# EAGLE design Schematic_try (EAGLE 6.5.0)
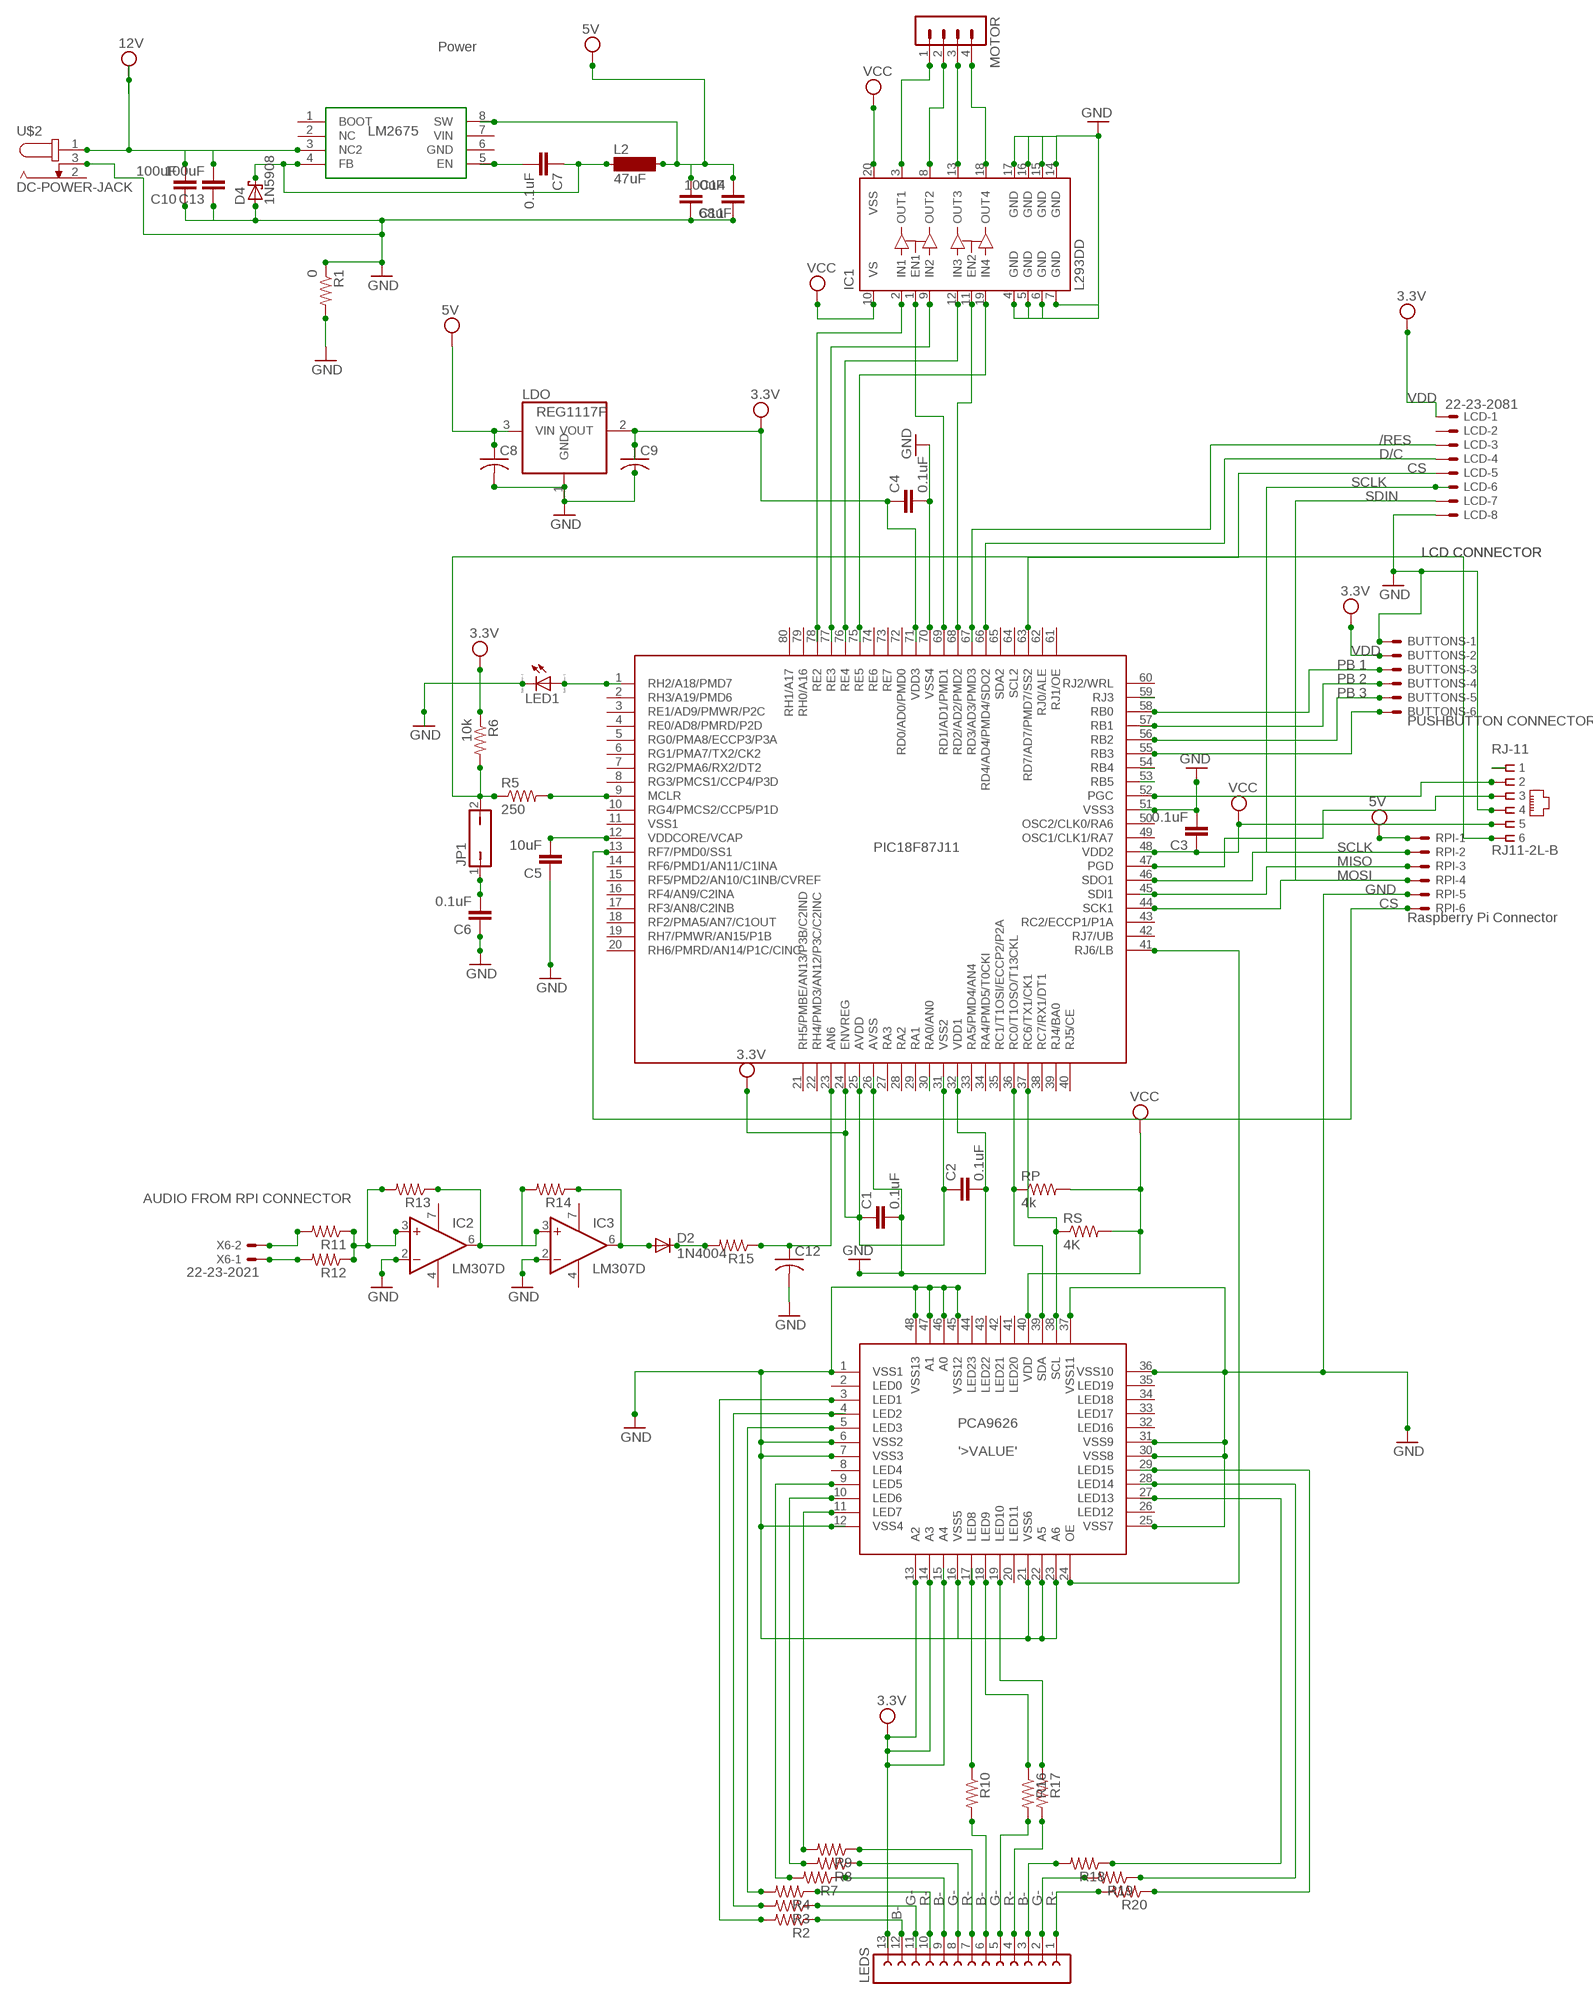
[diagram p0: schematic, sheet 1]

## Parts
BUTTONS  22-23-2061  [22-23-2061]
C1  0.1uF  C-EUC1206  [C1206]
C2  0.1uF  C-EUC1206  [C1206]
C3  0.1uF  C-EUC1206  [C1206]
C4  0.1uF  C-EUC1206  [C1206]
C5  10uF  C-EUC1206  [C1206]
C6  0.1uF  C-EUC1206  [C1206]
C7  0.1uF  C-EUC1206  [C1206]
C8  C-USC1206  [C1206]
C9  C-USC1206  [C1206]
C10  100uF  C-EUC1206  [C1206]
C11  100uF  C-EUC1206  [C1206]
C12  C-USC1206  [C1206]
C13  100uF  C-EUC1206  [C1206]
C14  68uF  C-EUC1206  [C1206]
D2  1N4004  [DO41-10]
D4  1N5908  [C4111-15]
IC1  L293DD  [SO20]
IC2  LM307D  [SO08]
IC3  LM307D  [SO08]
JP1  JP1Q  [JP1]
L2  47uF  SM-1206  [SM-1206]
LCD  22-23-2081  [22-23-2081]
LDO  REG1117F  [DD-3]
LED1  LED_E  [LED_1206]
LED_DRIVER  PCA9626  [SO-48/DIP]
LEDS  FE13-1  [FE13]
MOTOR  MA04-1  [MA04-1]
R1  0  R-US_R1206  [R1206]
R2  R-US_R1206  [R1206]
R3  R-US_R1206  [R1206]
R4  R-US_R1206  [R1206]
R5  250  R-US_R1206  [R1206]
R6  10k  R-US_R1206  [R1206]
R7  R-US_R1206  [R1206]
R8  R-US_R1206  [R1206]
R9  R-US_R1206  [R1206]
R10  R-US_R1206  [R1206]
R11  R-US_R1206  [R1206]
R12  R-US_R1206  [R1206]
R13  R-US_R1206  [R1206]
R14  R-US_R1206  [R1206]
R15  R-US_R1206  [R1206]
R16  R-US_R1206  [R1206]
R17  R-US_R1206  [R1206]
R18  R-US_R1206  [R1206]
R19  R-US_R1206  [R1206]
R20  R-US_R1206  [R1206]
RJ-11  RJ11-2L-B  [RJ11-NO_SHIELD]
RP  4k  R-US_R1206  [R1206]
RPI  22-23-2061  [22-23-2061]
RS  4K  R-US_R1206  [R1206]
U$1  PIC18F87J11  [S0-80/DIP]
U$2  DC-POWER-JACK  [PJ-036BH-SMT]
U$4  LM265  [8PIN]
X6  22-23-2021  [22-23-2021]

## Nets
+3.3: BUTTONS.2 C1.1 C2.1 C3.1 C4.1 C9.1 LCD.1 LDO.2(VOUT) LED_DRIVER.13(A2) LED_DRIVER.14(A3) LED_DRIVER.15(A4) LED_DRIVER.40(VDD) LEDS.13 R6.1 RJ-11.5 RP.2 RS.2 U$1.24(ENVREG) U$1.25(AVDD) U$1.31(VSS2) U$1.48(VDD2) U$1.71(VDD3) ; supply symbol labelled 3.3V, VCC
+5: C8.1 C11.2 C14.1 IC1.20(VSS) L2.2 LDO.3(VIN) RPI.1 U$4.8(SW) ; supply symbol labelled 5V, VCC
+12: C10.2 C13.2 IC1.10(VS) U$2.1 U$4.3(NC2) ; supply symbol labelled 12V, VCC
AGND: C12.2 IC2.2(-IN) IC3.2(-IN) R1.2 ; supply symbol labelled GND
GND: BUTTONS.1 C1.2 C2.2 C3.2 C4.2 C5.1 C6.1 C8.2 C10.1 C11.1 C13.1 C14.2 D4.A IC1.4(GND) IC1.5(GND) IC1.6(GND) IC1.7(GND) IC1.14(GND) IC1.15(GND) IC1.16(GND) IC1.17(GND) LCD.8 LDO.1(GND) LED1.C LED_DRIVER.1(VSS1) LED_DRIVER.6(VSS2) LED_DRIVER.7(VSS3) LED_DRIVER.12(VSS4) LED_DRIVER.16(VSS5) LED_DRIVER.21(VSS6) LED_DRIVER.22(A5) LED_DRIVER.23(A6) LED_DRIVER.25(VSS7) LED_DRIVER.30(VSS8) LED_DRIVER.31(VSS9) LED_DRIVER.36(VSS10) LED_DRIVER.37(VSS11) LED_DRIVER.45(VSS12) LED_DRIVER.46(A0) LED_DRIVER.47(A1) LED_DRIVER.48(VSS13) R1.1 RJ-11.4 RPI.5 U$1.26(AVSS) U$1.32(VDD1) U$1.51(VSS3) U$1.70(VSS4) U$2.3
N$1: LCD.7 RPI.4 U$1.44(SCK1)
N$2: RJ-11.3 U$1.47(PGD)
N$3: RPI.3 U$1.45(SDI1)
N$4: RJ-11.2 U$1.52(PGC)
N$5: LED1.A U$1.1(RH2/A18/PMD7)
N$6: C6.2 JP1.1
N$7: LED_DRIVER.24(OE) U$1.41(RJ6/LB)
N$9: LED_DRIVER.38(SCL) RS.1 U$1.37(RC6/TX1/CK1)
N$11: LED_DRIVER.5(LED3) R4.2
N$12: IC1.3(OUT1) MOTOR.1
N$13: IC1.8(OUT2) MOTOR.2
N$14: IC1.13(OUT3) MOTOR.3
N$15: IC1.18(OUT4) MOTOR.4
N$16: IC1.1(EN1)
N$17: IC1.9(IN2) U$1.77(RE3)
N$19: IC1.2(IN1) U$1.78(RE2)
N$20: IC1.11(EN2) U$1.68(RD2/AD2/PMD2)
N$21: U$1.69(RD1/AD1/PMD1)
N$25: LEDS.12 R2.1
N$26: U$1.59(RJ3)
N$27: C5.2 U$1.12(VDDCORE/VCAP)
N$28: JP1.2 R5.1 R6.2 RJ-11.6
N$29: R5.2 U$1.9(MCLR)
N$30: LEDS.11 R3.1
N$32: LED_DRIVER.4(LED2) R3.2
N$33: LCD.5 U$1.63(RD7/AD7/PMD7/SS2)
N$34: U$1.54(RB4)
N$36: LCD.3 U$1.67(RD3/AD3/PMD3)
N$37: LEDS.10 R4.1
N$39: U$1.53(RB5)
N$40: LEDS.9 R7.1
N$41: IC1.12(IN3) U$1.76(RE4)
N$42: LEDS.8 R8.1
N$43: LEDS.7 R9.1
N$44: LEDS.6 R10.2
N$45: LED_DRIVER.39(SDA) RP.1 U$1.36(RC0/T1OSO/T13CKL)
N$46: LED_DRIVER.29(LED15) R20.1
N$47: LED_DRIVER.28(LED14) R19.1
N$48: LED_DRIVER.27(LED13) R18.1
N$49: C7.1 D4.C L2.1 U$4.4(FB)
N$50: LED_DRIVER.19(LED10) R17.1
N$51: LED_DRIVER.18(LED9) R16.1
N$52: C7.2 U$4.5(EN)
N$53: LED_DRIVER.11(LED7) R9.2
N$54: LED_DRIVER.10(LED6) R8.2
N$55: LED_DRIVER.9(LED5) R7.2
N$56: RPI.6 U$1.13(RF7/PMD0/SS1)
N$57: U$1.30(RA0/AN0)
N$59: LED_DRIVER.17(LED8) R10.1
N$60: BUTTONS.4 U$1.57(RB1)
N$62: LEDS.5 R16.2
N$63: LCD.4 U$1.66(RD4/AD4/PMD4/SDO2)
N$64: LED_DRIVER.3(LED1) R2.2
N$65: LEDS.4 R17.2
N$66: LEDS.3 R18.2
N$67: LEDS.2 R19.2
N$68: LEDS.1 R20.2
N$69: RJ-11.1
N$70: IC1.19(IN4) U$1.75(RE5)
N$93: R11.2 X6.2
N$94: R12.2 X6.1
N$95: BUTTONS.3 U$1.58(RB0)
N$96: BUTTONS.5 U$1.56(RB2)
N$97: BUTTONS.6 U$1.55(RB3)
N$99: IC2.3(+IN) R11.1 R12.1 R13.2
N$100: IC2.6(OUT) IC3.3(+IN) R13.1 R14.2
N$101: D2.A IC3.6(OUT) R14.1
N$102: D2.C R15.2
N$103: C12.1 R15.1 U$1.23(AN6)
RPI: LCD.6 RPI.2 U$1.46(SDO1)
Unconnected: C9.2 LCD.2 LED_DRIVER.2(LED0) LED_DRIVER.8(LED4) LED_DRIVER.20(LED11) LED_DRIVER.26(LED12) LED_DRIVER.32(LED16) LED_DRIVER.33(LED17) LED_DRIVER.34(LED18) LED_DRIVER.35(LED19) LED_DRIVER.41(LED20) LED_DRIVER.42(LED21) LED_DRIVER.43(LED22) LED_DRIVER.44(LED23) U$1.2(RH3/A19/PMD6) U$1.3(RE1/AD9/PMWR/P2C) U$1.4(RE0/AD8/PMRD/P2D) U$1.5(RG0/PMA8/ECCP3/P3A) U$1.6(RG1/PMA7/TX2/CK2) U$1.7(RG2/PMA6/RX2/DT2) U$1.8(RG3/PMCS1/CCP4/P3D) U$1.10(RG4/PMCS2/CCP5/P1D) U$1.11(VSS1) U$1.14(RF6/PMD1/AN11/C1INA) U$1.15(RF5/PMD2/AN10/C1INB/CVREF) U$1.16(RF4/AN9/C2INA) U$1.17(RF3/AN8/C2INB) U$1.18(RF2/PMA5/AN7/C1OUT) U$1.19(RH7/PMWR/AN15/P1B) U$1.20(RH6/PMRD/AN14/P1C/CINC) U$1.21(RH5/PMBE/AN13/P3B/C2IND) U$1.22(RH4/PMD3/AN12/P3C/C2INC) U$1.27(RA3) U$1.28(RA2) U$1.29(RA1) U$1.33(RA5/PMD4/AN4) U$1.34(RA4/PMD5/T0CKI) U$1.35(RC1/T1OSI/ECCP2/P2A) U$1.38(RC7/RX1/DT1) U$1.39(RJ4/BA0) U$1.40(RJ5/CE) U$1.42(RJ7/UB) U$1.43(RC2/ECCP1/P1A) U$1.49(OSC1/CLK1/RA7) U$1.50(OSC2/CLK0/RA6) U$1.60(RJ2/WRL) U$1.61(RJ1/OE) U$1.62(RJ0/ALE) U$1.64(SCL2) U$1.65(SDA2) U$1.72(RD0/AD0/PMD0) U$1.73(RE7) U$1.74(RE6) U$1.79(RH0/A16) U$1.80(RH1/A17) U$2.2 U$4.1(BOOT) U$4.2(NC) U$4.6(GND) U$4.7(VIN)

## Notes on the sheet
- Power
- VDD
- /RES
- D/C
- CS
- SCLK
- SDIN
- LCD CONNECTOR | LCD CONNECTOR
- VDD
- PB 1
- PB 2
- PB 3
- PUSHBUTTON CONNECTOR
- SCLK
- MISO
- MOSI
- GND
- CS
- Raspberry Pi Connector
- AUDIO FROM RPI CONNECTOR
- G- | R- | B- | G- | R- | B- | G- | R- | B- | G- | R-
- B-

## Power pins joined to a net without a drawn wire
V+: IC2.7(V+) IC3.7(V+)
V-: IC2.4(V-) IC3.4(V-)

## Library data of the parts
BUTTONS RPI = con-molex:22-23-2061: .100" (2.54mm) Center Header - 6 Pin; MF: MOLEX; MPN: 22-23-2061; OC_FARNELL: 1462922; OC_NEWARK: 27C1933
C1-C7 C10 C11 C13 C14 = rcl:C-EU: CAPACITOR, European symbol
C8 C9 C12 = rcl:C-US: CAPACITOR, American symbol
D2 = diode:1N4004: DIODE
D4 = diode:1N5908: DIODE
IC1 = st-microelectronics:L293DD: PUSH-PULL FOUR CHANNEL DRIVER WITH DIODES Source: http://www.st.com/stonline/books/pdf/docs/1330.pdf; OC_FARNELL: unknown
IC2 IC3 = linear:LM307: OP AMP
JP1 = jumper:JP1Q: JUMPER
L2 = inductor-neosid:SM-1206: INDUCTOR; OC_FARNELL: unknown; OC_NEWARK: unknown
LCD = con-molex:22-23-2081: .100" (2.54mm) Center Header - 8 Pin; MF: MOLEX; MPN: 22-23-2081; OC_FARNELL: 1756826; OC_NEWARK: 01C7592
LDO = burr-brown:REG1117: 800mA and 1A Low Dropout (LDO) Positive Regulator 1.8V, 2.5V, 2.85V, 3.3V, 5V, and Adj; MF: TEXAS INSTRUMENTS; MPN: REG1117FAKTTT; OC_FARNELL: 1296120; OC_NEWARK: 87H2562
LED1 = eagle-ltspice:LED_E: LED; SPICEMODEL: NONE; SPICEPREFIX: D; SPICETYPE: diode
LED_DRIVER = PCA9626:PCA9626
LEDS = con-lsta:FE13-1: FEMALE HEADER; OC_FARNELL: unknown; OC_NEWARK: unknown
MOTOR = con-lstb:MA04-1: PIN HEADER; OC_FARNELL: unknown; OC_NEWARK: unknown
R1-R20 RP RS = resistor:R-US_: RESISTOR, American symbol
RJ-11 = con-tycoelectronics:RJ11: CORCOM Modular RJ Jacks No Shield Source: www.tycoelectronics.com .. ENG_DS_1654001_1099_RJ_L_0507.pdf; MF: TYCO ELECTRONICS; MPN: RJ11-2L-B; OC_FARNELL: unknown; OC_NEWARK: 83F4463
U$1 = PIC18F87J11:PIC18F87J11
U$2 = PJ-036BH-SMT:DC-POWER-JACK
U$4 = LM2675:LM265
X6 = con-molex:22-23-2021: .100" (2.54mm) Center Header - 2 Pin; MF: MOLEX; MPN: 22-23-2021; OC_FARNELL: 1462926; OC_NEWARK: 25C3832

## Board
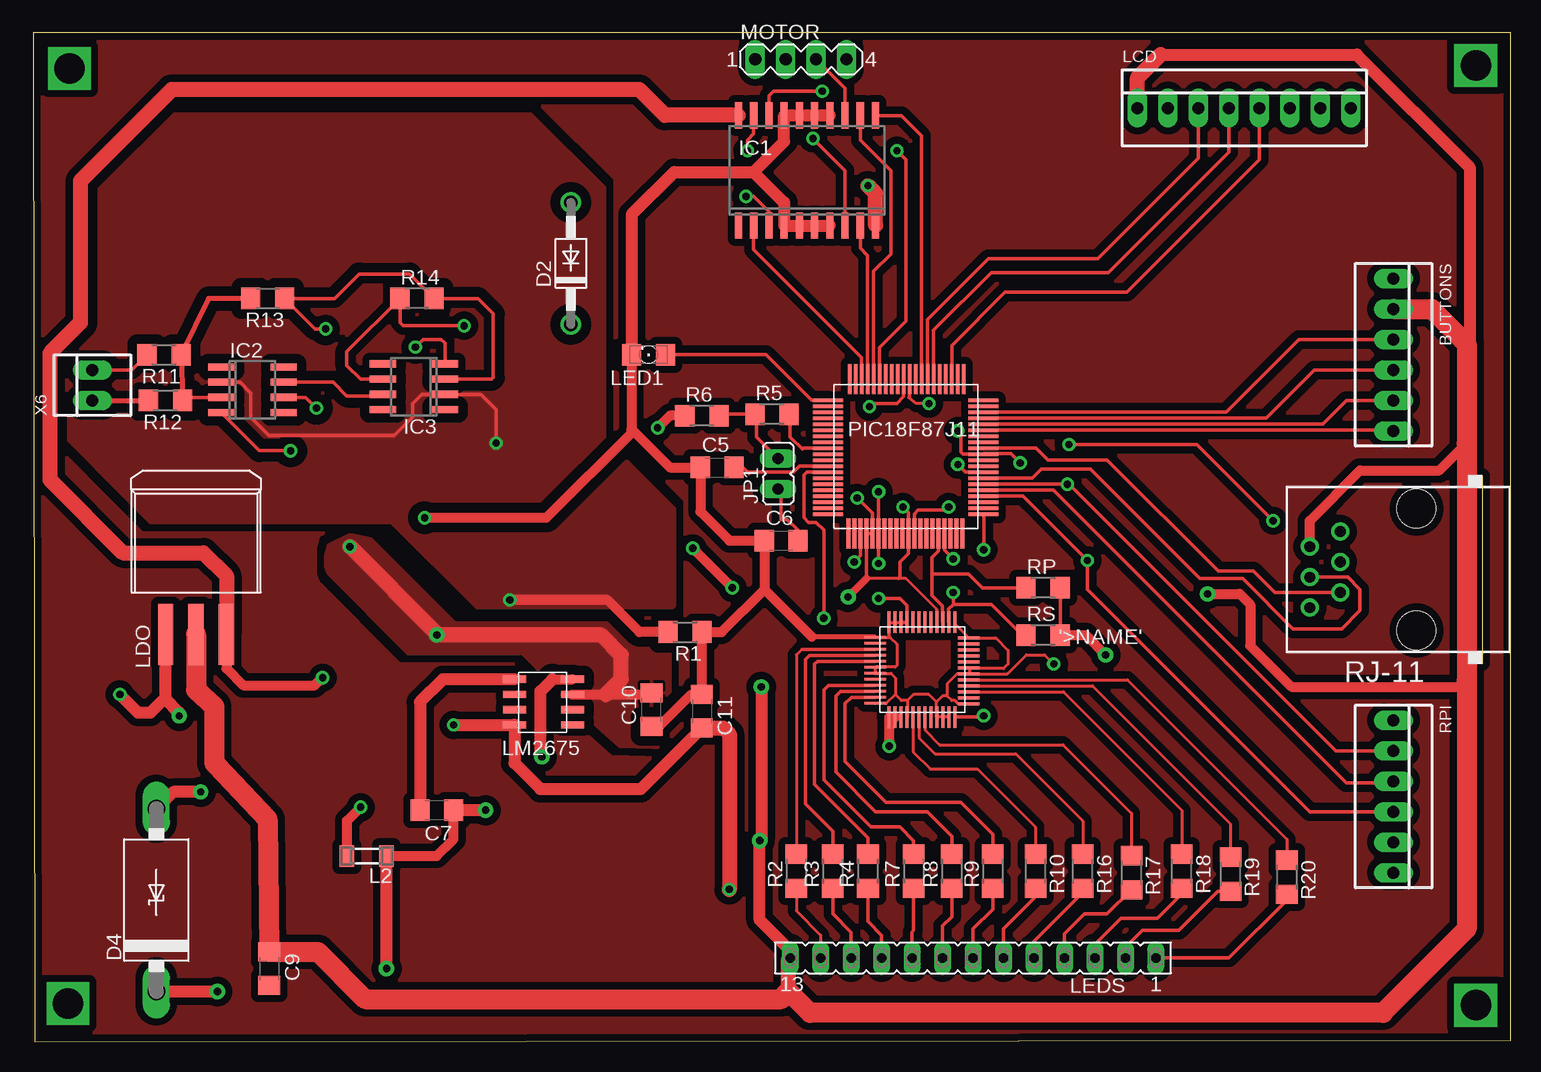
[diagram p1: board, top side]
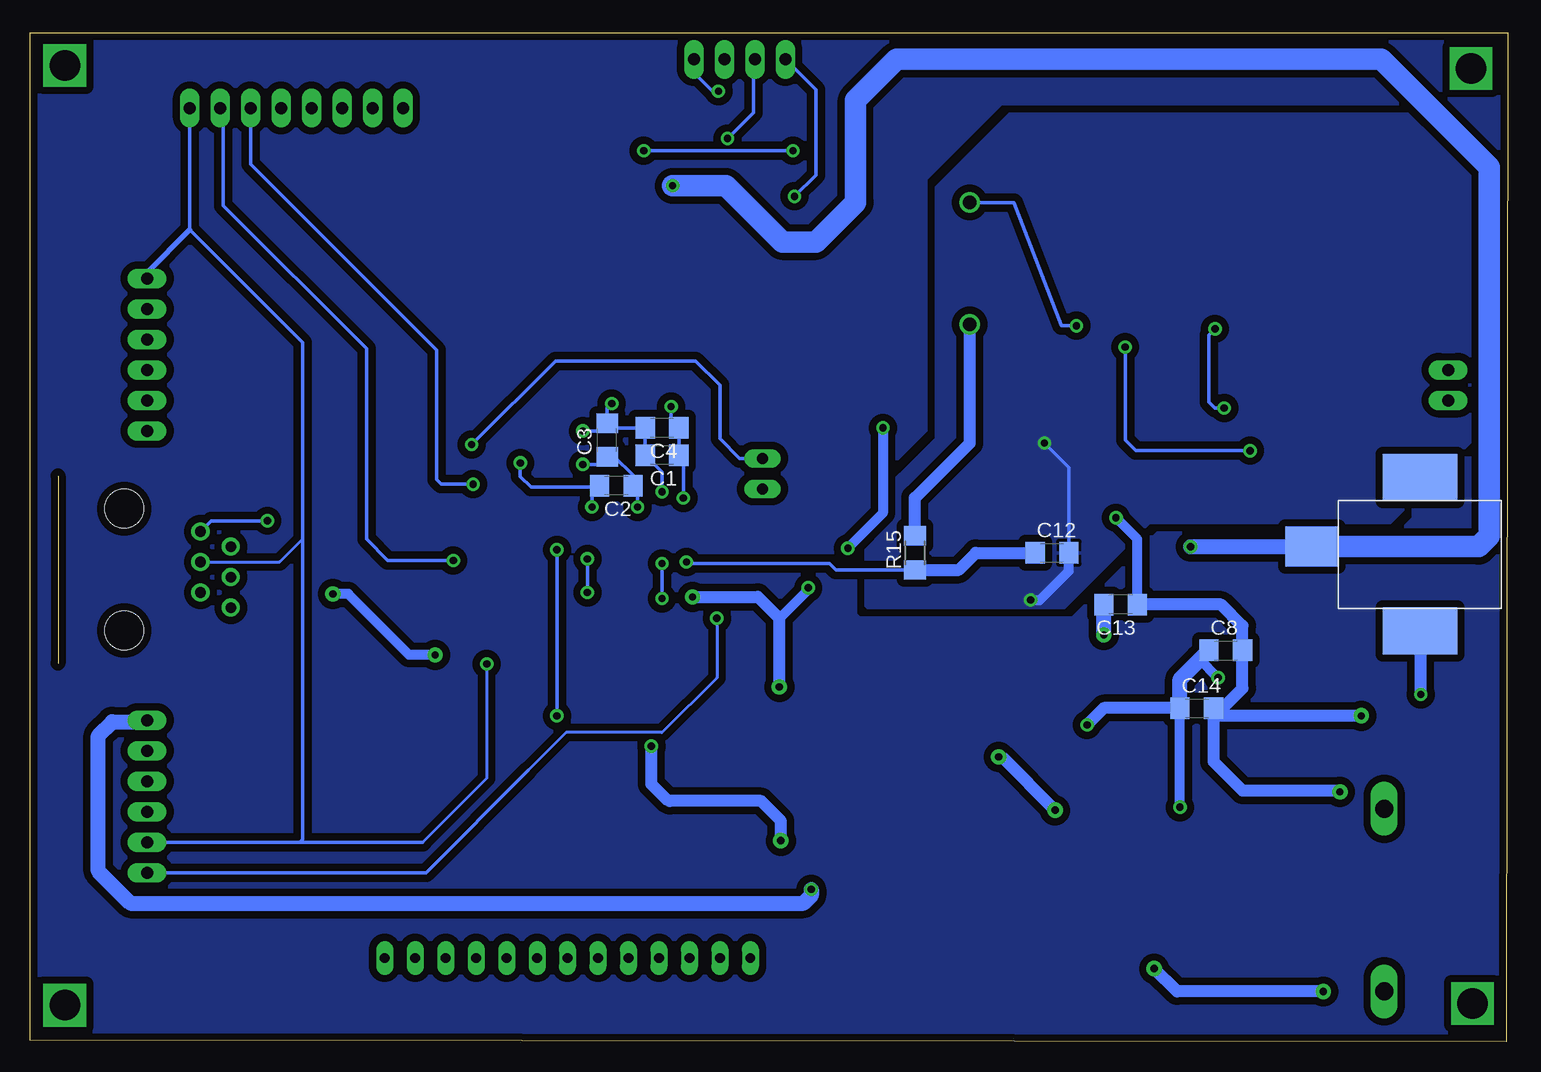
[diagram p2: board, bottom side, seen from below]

Size 123.17 x 84.12 mm. Coordinates in mm from the lower left corner, seen from the top.
Outline: 0.13,0 123.17,0.13 123.17,84.12 0,84.12 0.13,0
Copper layers (1*16): Top 0.035mm / dielectric 1.5mm / Bottom 0.035mm
Design rules "SparkFunDRC": minimum track width 8mil, minimum drill 20mil, track to track 8mil, track to pad 8mil, pad to pad 8mil, via to via 8mil, smd to smd 8mil, copper to edge 10mil, drill to drill 8mil, minimum pad ring 12mil, minimum via ring 10mil, stop-mask expansion 4mil, vias tented up to drill 25mil, thermal gap 10mil

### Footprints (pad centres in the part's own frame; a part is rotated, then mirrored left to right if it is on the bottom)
22-23-2061 = drill 1 long: 1 -6.35,0; 2 -3.81,0; 3 -1.27,0; 4 1.27,0; 5 3.81,0; 6 6.35,0
C1206 = smd 1.6 x 1.8: 1 -1.4,0; 2 1.4,0
DO41-10 = drill 1.118: A 5.08,0; C -5.08,0
C4111-15 = drill 1.499 long: A 7.62,0; C -7.62,0
SO20 = smd 0.6 x 2.2: 1 -5.715,-4.6; 2 -4.445,-4.6; 3 -3.175,-4.6; 4 -1.905,-4.6; 5 -0.635,-4.6; 6 0.635,-4.6; 7 1.905,-4.6; 8 3.175,-4.6; 9 4.445,-4.6; 10 5.715,-4.6; 11 5.715,4.6; 12 4.445,4.6; 13 3.175,4.6; 14 1.905,4.6; 15 0.635,4.6; 16 -0.635,4.6; 17 -1.905,4.6; 18 -3.175,4.6; 19 -4.445,4.6; 20 -5.715,4.6
SO08 = smd 0.6 x 2.2: 1 -1.905,-2.6; 2 -0.635,-2.6; 3 0.635,-2.6; 4 1.905,-2.6; 5 1.905,2.6; 6 0.635,2.6; 7 -0.635,2.6; 8 -1.905,2.6
JP1 = drill 0.914 long: 1 0,-1.27; 2 0,1.27
SM-1206 = smd 1.2 x 1.8: 1 -1.65,0; 2 1.65,0
22-23-2081 = drill 1 long: 1 -8.89,0; 2 -6.35,0; 3 -3.81,0; 4 -1.27,0; 5 1.27,0; 6 3.81,0; 7 6.35,0; 8 8.89,0
DD-3 = smd 1.27 x 5.08: 1 -2.54,-7.938; 2 0,-7.938; 3 2.54,-7.938
LED_1206 = smd 1.6 x 1.803: A -1.422,0; C 1.422,0
SO-48/DIP = smd 1.8 x 0.22: 1 -7.65,5.65; 2 -7.65,5.15; 3 -7.65,4.65; 4 -7.65,4.15; 5 -7.65,3.65; 6 -7.65,3.15; 7 -7.65,2.65; 8 -7.65,2.15; 9 -7.65,1.65; 10 -7.65,1.15; 11 -7.65,0.65; 12 -7.65,0.15; 25 0.15,0.1; 26 0.15,0.6; 27 0.15,1.1; 28 0.15,1.6; 29 0.15,2.1; 30 0.15,2.6; 31 0.15,3.1; 32 0.15,3.6; 33 0.15,4.1; 34 0.15,4.6; 35 0.15,5.1; 36 0.15,5.6 | smd 0.22 x 1.8: 13 -6.5,-1; 14 -6,-1; 15 -5.5,-1; 16 -5,-1; 17 -4.5,-1; 18 -4,-1; 19 -3.5,-1; 20 -3,-1; 21 -2.5,-1; 22 -2,-1; 23 -1.5,-1; 24 -1,-1; 37 -1,6.9; 38 -1.5,6.9; 39 -2,6.9; 40 -2.5,6.9; 41 -3,6.9; 42 -3.5,6.9; 43 -4,6.9; 44 -4.5,6.9; 45 -5,6.9; 46 -5.5,6.9; 47 -6,6.9; 48 -6.5,6.9
FE13 = drill 0.813 long: 1 -15.24,0; 2 -12.7,0; 3 -10.16,0; 4 -7.62,0; 5 -5.08,0; 6 -2.54,0; 7 0,0; 8 2.54,0; 9 5.08,0; 10 7.62,0; 11 10.16,0; 12 12.7,0; 13 15.24,0
MA04-1 = drill 1.016 long: 1 -3.81,0; 2 -1.27,0; 3 1.27,0; 4 3.81,0
R1206 = smd 1.6 x 1.803: 1 -1.422,0; 2 1.422,0
RJ11-NO_SHIELD = drill 0.9 pad 1.4: 1 -3.175,8.89; 2 -1.905,6.35; 3 -0.635,8.89; 4 0.635,6.35; 5 1.905,8.89; 6 3.175,6.35 | hole 3.251: -5.08,0; 5.08,0
S0-80/DIP = smd 2.5 x 0.3: 1 -7,11.2; 2 -7,10.7; 3 -7,10.2; 4 -7,9.7; 5 -7,9.2; 6 -7,8.7; 7 -7,8.2; 8 -7,7.7; 9 -7,7.2; 10 -7,6.7; 11 -7,6.2; 12 -7,5.7; 13 -7,5.2; 14 -7,4.7; 15 -7,4.2; 16 -7,3.7; 17 -7,3.2; 18 -7,2.7; 19 -7,2.2; 20 -7,1.7; 41 5.95,1.7; 42 5.95,2.2; 43 5.95,2.7; 44 5.95,3.2; 45 5.95,3.7; 46 5.95,4.2; 47 5.95,4.7; 48 5.95,5.2; 49 5.95,5.7; 50 5.95,6.2; 51 5.95,6.7; 52 5.95,7.2; 53 5.95,7.7; 54 5.95,8.2; 55 5.95,8.7; 56 5.95,9.2; 57 5.95,9.7; 58 5.95,10.2; 59 5.95,10.7; 60 5.95,11.2 | smd 0.3 x 2.5: 21 -5.3,0.1; 22 -4.8,0.1; 23 -4.3,0.1; 24 -3.8,0.1; 25 -3.3,0.1; 26 -2.8,0.1; 27 -2.3,0.1; 28 -1.8,0.1; 29 -1.3,0.1; 30 -0.8,0.1; 31 -0.3,0.1; 32 0.2,0.1; 33 0.7,0.1; 34 1.2,0.1; 35 1.7,0.1; 36 2.2,0.1; 37 2.7,0.1; 38 3.2,0.1; 39 3.7,0.1; 40 4.2,0.1; 61 4.3,12.95; 62 3.8,12.95; 63 3.3,12.95; 64 2.8,12.95; 65 2.3,12.95; 66 1.8,12.95; 67 1.3,12.95; 68 0.8,12.95; 69 0.3,12.95; 70 -0.2,12.95; 71 -0.7,12.95; 72 -1.2,12.95; 73 -1.7,12.95; 74 -2.2,12.95; 75 -2.7,12.95; 76 -3.2,12.95; 77 -3.7,12.95; 78 -4.2,12.95; 79 -4.7,12.95; 80 -5.2,12.95
PJ-036BH-SMT = smd 4.4 x 3.3: 1 15.8,-0.65 | smd 6.2 x 3.9: 2 6.8,-6.4; 3 6.8,6.4
8PIN = smd 1.91 x 0.6: 1 -8.89,3.81; 2 -8.89,2.54; 3 -8.89,1.27; 4 -8.89,0; 5 -4.06,0; 6 -4.06,1.27; 7 -4.06,2.54; 8 -4.06,3.81
22-23-2021 = drill 1 long: 1 -1.27,0; 2 1.27,0

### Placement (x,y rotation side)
BUTTONS  113.41,57.28 270 top
C1  70.49,48.89 180 bottom
C2  74.29,46.35 180 bottom
C3  75.06,50.16 90 bottom
C4  70.49,51.18 180 bottom
C5  57.02,47.88 0 top
C6  62.36,41.78 0 top
C7  33.65,19.3 180 top
C8  23.49,32.64 0 bottom
C9  19.69,6.1 270 top
C10  51.56,27.69 90 top
C11  55.75,27.56 270 top
C12  37.97,40.77 0 bottom
C13  32.26,36.45 180 bottom
C14  25.91,27.81 0 bottom
D2  44.83,64.9 90 top
D4  10.29,11.81 90 top
IC1  64.52,72.64 0 top
IC2  18.29,54.36 270 top
IC3  31.75,54.61 90 top
JP1  62.1,47.37 0 top
L2  27.81,15.49 180 top
LCD  100.97,77.85 0 top
LDO  13.59,41.91 0 top
LED1  51.31,57.28 180 top
LED_DRIVER  77.85,28.07 0 top
LEDS  78.36,6.98 180 top
MOTOR  64.01,81.91 0 top
R1  54.36,34.16 180 top
R2  63.63,14.22 90 top
R3  66.68,14.22 90 top
R4  69.6,14.22 90 top
R5  61.6,52.32 0 top
R6  55.75,52.2 0 top
R7  73.41,14.22 90 top
R8  76.58,14.22 90 top
R9  80.01,14.22 90 top
R10  83.57,14.22 270 top
R11  10.92,57.28 180 top
R12  11.05,53.47 180 top
R13  19.56,61.98 180 top
R14  32,61.98 0 top
R15  49.4,40.77 90 bottom
R16  87.5,14.22 270 top
R17  91.57,14.1 270 top
R18  95.76,14.22 270 top
R19  99.82,13.97 270 top
R20  104.52,13.72 270 top
RJ-11  115.32,39.37 90 top
RP  84.2,37.85 0 top
RPI  113.41,20.45 270 top
RS  84.2,33.91 0 top
U$1  73.28,42.29 0 top
U$2  0.51,40.64 180 bottom
U$4  36.07,30.23 180 top
X6  4.95,54.74 90 top

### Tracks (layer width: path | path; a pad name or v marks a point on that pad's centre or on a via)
+3.3  (via drill 0.6, 0.6 pad 1.27)
  Top 0.254: LED_DRIVER.40 75.35,36.03 72.77,38.61 72.14,38.61 69.73,38.61 69.48,38.86 | 63.12,7.62 LEDS.13 62.99,6.86
  Top 0.305: 15.11,23.24 15.24,23.11 | 113.54,60.96 BUTTONS.2 | 69.48,38.62 69.48,38.86 U$1.24 U$1.25 69.98,44.07 v68.71,45.34 | 60.71,16.89 v60.58,16.76 | 119,29.59 119.51,30.1 | 71.37,27.04 LED_DRIVER.13 | LED_DRIVER.14 LED_DRIVER.15 | RP.2 RS.2 | U$1.48 77.73,47.49 v77.09,48.13 | v69.72,52.96 69.98,53.21 72.01,53.21 72.58,53.78 U$1.71 | 72.14,38.61 72.26,38.73 72.26,40 72.98,40.72 U$1.31 72.98,44.11 v72.52,44.58
  Top 0.61: 69.48,38.62 v67.94,37.08
  Top 0.813: v71.37,24.64 71.37,27.04 | v89.41,32.26 87.76,33.91 RS.2 | 119,29.59 104.9,29.59 101.47,33.02 101.47,36.45 100.58,37.34 v97.92,37.34 | LED_DRIVER.13 LED_DRIVER.14 | RJ-11.5 106.43,43.43 110.62,47.62 117.22,47.62 119.51,49.91 | R6.1 53.09,52.2 v52.07,51.18 | v54.99,41.15 v58.29,37.85
  Top 1.016: v60.58,16.76 60.58,10.16 63.12,7.62 | v60.71,29.59 60.71,16.89 | 93.98,82.3 110.36,82.3 119.76,72.9 119.76,58.42 119.51,58.17
  Top 1.27: LCD.1 92.07,80.39 93.98,82.3 | 119.63,59.05 119.13,58.55 | 62.99,4.19 62.99,6.86
  Top 1.676: LDO.2 13.59,29.34 15.11,27.94 15.11,23.24 | 15.24,23.11 19.56,18.54 C9.1 23.75,7.5 27.69,3.56 62.36,3.56 62.99,4.19 64.77,2.41 112.52,2.41 119.51,9.4 119.51,30.1 119.51,49.91 119.51,58.17 119.13,58.55 116.59,61.09 BUTTONS.2
  Bottom 0.254: 69.98,19.94 70.1,19.94 70.1,20.19
  Bottom 0.305: 69.85,20.07 69.98,19.94 | v68.71,45.34 68.71,48.52 C1.1 C4.1 69.72,51.82 v69.72,52.96 | 72.52,45.47 C2.1 | v77.09,48.13 75.69,48.13 C3.1 74.42,48.77 72.9,47.24 C2.1 | v72.52,44.58 72.52,45.98 C2.1
  Bottom 0.406: v58.29,37.85 58.29,37.72
  Bottom 0.813: v97.92,37.34 96.65,37.34 91.57,32.26 v89.41,32.26 | v52.07,51.18 52.07,44.07 v54.99,41.15 | 58.29,37.72 60.71,35.31
  Bottom 1.016: v60.58,16.76 60.58,18.42 62.23,20.07 69.85,20.07 | v67.94,37.08 62.48,37.08 60.71,35.31 v60.71,29.59 | 70.1,20.19 71.37,21.46 v71.37,24.64
+5  (via drill 0.6)
  Top 0.305: U$4.8 40.13,26.29
  Top 0.813: LDO.3 16.13,31.11 17.53,29.72 23.49,29.72 v24.13,30.35 | L2.2 26.16,18.42 v27.3,19.56
  Top 1.016: v35.05,26.42 U$4.8 40.13,23.25 42.29,21.08 50.68,21.08 C11.2
  Top 1.27: IC1.20 52.68,77.24 50.55,79.38 11.56,79.38 3.94,71.75 3.94,59.94 1.4,57.4 1.4,46.86 7.49,40.77 14.22,40.77 16.13,38.86 LDO.3 | C11.2 57.53,26.16 58.04,25.65 v58.04,12.7
  Bottom 0.305: 113.54,26.67 RPI.1
  Bottom 0.813: v24.13,30.35 25.65,31.88 | v27.3,19.56 C14.1
  Bottom 1.016: C14.1 33.65,27.81 v35.05,26.42
  Bottom 1.27: C14.1 27.31,30.23 25.65,31.88 C8.1 | 113.54,26.67 116.33,26.67 117.47,25.53 117.47,14.22 114.81,11.56 58.67,11.56 58.04,12.19 v58.04,12.7
+12  (via drill 0.6, 0.6 pad 1.27)
  Top 0.305: v33.65,33.91 33.65,34.04
  Top 0.813: 47.75,28.96 U$4.3 51.43,28.96 C10.2
  Top 1.27: 47.75,28.96 49.02,30.23 49.02,32.26 47.37,33.91 v33.65,33.91 | 33.65,34.04 v26.42,41.27 | IC1.10 70.23,70.74 v69.6,71.37
  Bottom 1.27: v33.65,33.91 C13.2 | v26.42,41.27 16.32,41.27 U$2.1
  Bottom 1.778: v69.6,71.37 65.15,71.37 60.45,66.67 57.66,66.67 54.36,69.98 54.36,78.49 50.93,81.91 10.54,81.91 1.52,72.9 1.52,42.16 2.41,41.27 16.29,41.27 U$2.1
  pour Top (isolate 0.813): 24.64,38.99 31.24,32.39 40.77,32.39 42.93,30.23 44.45,28.57 48.9,24.64 52.96,24.51 53.09,29.72 53.09,33.02 52.96,33.15 52.96,33.53 51.56,34.92 35.18,34.92 28.19,41.91 26.42,42.29 24.64,41.4 24.38,40.51 24.38,39.62
AGND  (via drill 0.6)
  Top 0.305: v38.61,49.91 38.61,52.7 37.34,53.97 IC3.2 32.38,53.97 31.62,53.21 31.62,52.07 30.1,50.55 19.69,50.55 18.16,52.07 18.16,54.1 17.27,54.99 IC2.2
  Top 0.813: R1.2 50.55,34.16 47.88,36.83 v39.75,36.83
  Bottom 0.305: C12.2 36.57,47.88 v38.61,49.91
  Bottom 0.813: v39.75,36.83 38.99,36.83 36.58,39.24 C12.2
  pour Bottom (isolate 0.61, rank 4): 1.91,77.34 41.53,77.34 47.63,71.25 47.63,50.29 53.47,44.45 53.47,36.32 53.34,36.19 36.96,36.19 29.85,43.31 9.78,43.31 0.76,52.32 0.76,76.2
  pour Top (isolate 0.813): 0.76,76.2 1.91,77.34 41.53,77.34 47.63,71.25 47.63,50.29 53.47,44.45 53.47,36.32 53.34,36.19 36.96,36.19 36.83,36.32 29.85,43.31 9.78,43.31 0.76,52.32
GND  (via drill 0.6, 0.6 pad 0.25, 0.6 pad 1.02, 0.6 pad 1.27)
  Top 0.254: 70.14,33.78 LED_DRIVER.1 71.25,33.72 71.44,33.72 72.01,33.15 72.01,31.37 71.88,31.24 70.23,31.24 LED_DRIVER.6 LED_DRIVER.7 71.52,30.72 71.88,30.35 71.88,28.96 | 78.05,31.11 80.9,31.11 81.28,31.5 81.28,32.64 80.25,33.67 LED_DRIVER.36 76.85,34.82 LED_DRIVER.37 | 78.05,31.11 LED_DRIVER.31 | LED_DRIVER.30 81.21,30.67 82.8,32.26 84.33,32.26 v85.09,31.5 | 78.05,31.11 78.05,30.72 LED_DRIVER.30 | 75.31,28.32 75.31,27.03 LED_DRIVER.21 LED_DRIVER.22 LED_DRIVER.23 | 75.31,28.32 74.68,28.96 73.41,28.96 72.9,28.45 | 72.9,28.45 72.9,27.11 LED_DRIVER.16 | 71.88,28.96 71.12,28.19 70.22,28.19 LED_DRIVER.12 | 72.9,28.45 72.39,28.45 71.88,28.96 | LED_DRIVER.48 LED_DRIVER.47 LED_DRIVER.46 | 76.2,28.83 75.82,28.83 75.31,28.32 | LED_DRIVER.30 77.02,30.67 76.2,29.85 76.2,28.83 | LED_DRIVER.25 77.12,28.17 76.84,28.45 76.58,28.45 76.2,28.83 | v74.68,53.21 73.66,53.21 73.03,53.72
  Top 0.305: v13.97,20.83 13.95,20.83 | v12.19,27.18 12.19,27.43 | LED_DRIVER.46 LED_DRIVER.45 72.85,36.37 72.26,36.96 v70.49,36.96 | LED_DRIVER.48 71.35,33.82 71.25,33.72 | v76.33,44.58 76.07,44.32 73.79,44.32 73.48,44.02 U$1.32 | v77.09,50.93 77.34,50.67 77.34,49.15 77.5,48.99 U$1.51 79.26,49.02 81.53,49.02 v82.3,48.26 | v70.49,39.88 U$1.26 v70.48,45.84 v70.49,45.85 | 49.89,51.08 50.04,50.93 | LDO.1 11.05,28.7 | 73.03,53.72 73.08,53.72 U$1.70
  Top 0.406: 64.9,33.78 70.14,33.78 | C11.1 | 55.75,34.14 R1.1
  Top 0.813: 60.96,37.72 C6.1 58.04,41.78 55.62,44.2 C5.1 53.09,47.88 50.04,50.93 42.8,43.69 v32.64,43.69 | 60.96,37.72 64.9,33.78 | LED1.C 49.89,51.08 | C10.1 52.19,26.29 54.86,28.96 C11.1 | C11.1 55.75,34.14 | R1.1 57.4,34.16 60.96,37.72
  Top 1.016: v13.97,20.83 11.68,20.83 D4.A | 12.19,27.43 11.05,28.57 LDO.1 | LED1.C 49.91,57.3 49.91,68.96 53.47,72.52 60.07,72.52 | 60.07,72.52 62.61,69.98 IC1.4 IC1.5 IC1.6 IC1.7 | 60.07,72.52 62.61,75.06 IC1.17 IC1.16 IC1.15 IC1.14 | 11.05,28.7 9.78,27.43 8.76,27.43 v7.24,28.96
  Bottom 0.254: 90.42,16.64 85.09,21.97 v85.09,31.5 | RJ-11.4 102.36,40 100.46,41.91
  Bottom 0.305: 90.42,16.64 100.71,16.64 | 100.71,16.64 112.65,16.64 113.03,16.26 RPI.5 | 100.71,16.64 100.46,16.89 100.46,41.91 100.46,58.29 109.85,67.69 LCD.8 | 14.1,20.96 v13.97,20.83 | 23.75,27.81 C14.2 23.87,27.18 | C8.2 | v76.33,44.58 76.33,46.23 | v77.09,50.93 75.19,50.93 C3.2 | C3.2 74.67,51.18 C4.2 C1.2 70.49,47.49 v70.49,45.85 | 76.33,46.23 81.41,46.23 82.3,47.12 v82.3,48.26 | C3.2 75.06,52.83 v74.68,53.21 | v70.49,36.96 v70.49,39.88 | 76.33,46.23 75.82,46.23 C2.2 | 7.24,34.17 U$2.3
  Bottom 0.406: BUTTONS.1 113.41,64.13 109.85,67.69
  Bottom 0.813: C13.1 30.86,41.91 v32.64,43.69
  Bottom 1.016: C14.2 24.51,23.36 22.1,20.96 14.1,20.96 | 23.75,27.81 22.1,29.46 C8.2 | C8.2 22.1,34.67 23.88,36.45 C13.1 | v12.19,27.18 23.87,27.18 | v7.24,28.96 7.24,34.17
N$1  (via drill 0.6 pad 0.25)
  Top 0.305: U$1.44 82.53,45.49 v87.88,40.13 87.88,37.72 106.43,19.18 RPI.4
  Bottom 0.305: v87.88,40.13 93.34,40.13 95.12,41.91 95.12,57.78 107.06,69.72 107.06,77.6 LCD.7
N$2
  Top 0.305: U$1.47 83.31,46.99 84.07,47.75 88.14,47.75 97.28,38.61 100.84,38.61 105.03,34.42 109.09,34.42 110.62,35.94 110.62,37.72 109.6,38.73 RJ-11.3
N$3
  Top 0.305: U$1.45 85.07,45.99 109.47,21.59 113.28,21.59 RPI.3
N$4
  Top 0.305: U$1.52 83.6,49.49 84.58,48.51 89.53,48.51 98.81,39.24 101.73,39.24 103.5,37.47 RJ-11.2
N$5
  Top 0.305: U$1.1 64.87,53.49 61.09,57.28 LED1.A
N$6
  Top 0.305: C6.2 63.76,42.67 62.87,43.56 62.36,43.56 62.36,45.34 JP1.1
N$7  (via drill 0.6 pad 1.02)
  Top 0.305: LED_DRIVER.24 79.14,27.07 v79.25,27.18 | v79.25,41.02 79.25,43.97 U$1.41
  Bottom 0.305: v79.25,27.18 v79.25,41.02
N$9  (via drill 0.6 pad 1.02)
  Top 0.305: v76.71,37.47 76.71,36.45 | 76.71,36.45 76.33,36.07 76.33,34.99 LED_DRIVER.38 | RS.1 82.42,33.91 79.88,36.45 76.71,36.45 | U$1.37 75.98,40.99 v76.71,40.26
  Bottom 0.305: v76.71,40.26 v76.71,37.47
N$11
  Top 0.305: LED_DRIVER.5 65.37,31.72 65.15,31.5 65.15,21.46 69.6,17.02 R4.2
N$12  (via drill 0.6)
  Top 0.305: IC1.3 61.34,69.21 60.07,70.48 v59.44,70.48
  Bottom 0.305: v59.44,70.48 57.66,72.26 57.66,79.38 MOTOR.1
N$13  (via drill 0.6)
  Top 0.305: IC1.8 67.69,72.64 v65.02,75.31
  Bottom 0.305: v65.02,75.31 62.87,77.47 62.87,81.79 MOTOR.2
N$14
  Top 0.305: IC1.13 67.69,79.5 MOTOR.3
N$15  (via drill 0.6)
  Top 0.305: IC1.18 61.34,78.87 61.72,79.25 v65.79,79.25
  Bottom 0.305: v65.79,79.25 66.29,79.25 67.82,80.77 MOTOR.4
N$17
  Top 0.305: U$1.77 69.58,65.55 68.96,66.17 IC1.9
N$19
  Top 0.305: U$1.78 69.08,57.03 60.07,66.04 IC1.2
N$20
  Top 0.305: U$1.68 74.08,75.53 72.39,77.22 70.26,77.22 IC1.11
N$22
  pour Bottom (isolate 0.61, rank 6): 0.38,81.41 2.54,83.57 119.76,83.57 122.68,80.64 122.68,2.54 120.65,0.51 3.17,0.51 0.51,3.18 0.38,3.3
N$23
  pour Top (isolate 0.61, rank 6): 0.38,81.41 2.54,83.57 119.76,83.57 122.68,80.64 122.68,2.54 120.65,0.51 3.17,0.51 0.38,3.3
N$25
  Top 0.254: R2.1 63.63,10.92 65.66,8.89 LEDS.12
N$27
  Top 0.305: C5.2 59.07,47.99 59.31,47.75 59.57,47.5 | U$1.12 64.15,47.99 64.13,48.01 63.88,48.01 63.37,47.5 59.57,47.5 | 59.69,47.37 59.57,47.5
N$28  (via drill 0.6)
  Top 0.305: JP1.2 60.32,50.42 60.32,52.17 R5.1 57.3,52.32 R6.2 | v86.36,49.78 97.03,49.78 v103.38,43.43
  Bottom 0.305: JP1.2 64.01,48.64 65.66,50.29 65.66,54.74 67.69,56.77 79.38,56.77 v86.36,49.78 | v103.38,43.43 108.08,43.43 RJ-11.6
N$29
  Top 0.305: U$1.9 64.22,49.49 64.13,49.4 63.12,50.42 63.12,52.22 R5.2
N$30
  Top 0.305: R3.1 66.68,10.67 68.2,9.14 LEDS.11
N$32
  Top 0.305: LED_DRIVER.4 64.73,32.22 64.39,31.88 64.39,19.81 66.68,17.53 R3.2
N$33
  Top 0.305: U$1.63 76.58,58.04 81.03,62.48 91.19,62.48 102.23,73.53 LCD.5
N$35  (via drill 2.54)
  other vias: 3.05,81.15
N$36
  Top 0.305: U$1.67 74.58,60.23 79.63,65.28 88.77,65.28 97.16,73.66 LCD.3
N$37
  Top 0.305: R4.1 69.6,10.03 70.74,8.89 LEDS.10
N$38  (via drill 2.54)
  other vias: 120.27,81.41
N$40
  Top 0.305: R7.1 73.41,9.27 73.28,9.14 LEDS.9
N$41
  Top 0.305: U$1.76 70.08,64.24 71.5,65.66 71.5,72.64 68.96,75.18 IC1.12
N$42
  Top 0.305: R8.1 76.58,10.41 75.82,9.65 LEDS.8
N$43
  Top 0.305: R9.1 80.01,11.05 78.36,9.4 LEDS.7
N$44
  Top 0.305: R10.2 83.57,12.07 80.9,9.4 LEDS.6
N$45
  Top 0.305: U$1.36 75.48,40.94 74.93,40.39 74.93,38.99 | 74.93,38.99 74.93,37.21 75.82,36.32 75.82,35 LED_DRIVER.39 | RP.1 79.12,37.85 77.98,38.99 74.93,38.99
N$46
  Top 0.254: LED_DRIVER.29 91.25,30.17 104.52,16.89 R20.1
N$47
  Top 0.254: LED_DRIVER.28 88.32,29.67 99.82,18.16 R19.1
N$48
  Top 0.254: LED_DRIVER.27 85.89,29.17 95.76,19.3 R18.1
N$49  (via drill 0.6 pad 1.27)
  Top 0.305: 42.29,23.88 v42.42,23.75
  Top 0.813: 43.31,30.23 U$4.4 | L2.1 33.65,15.49 35.05,16.89 C7.1
  Top 1.016: D4.C v15.37,4.19 | v29.46,6.1 29.46,10.92 L2.1 | v37.72,19.3 C7.1 | 42.29,23.88 42.29,29.21 43.31,30.23
  Bottom 0.305: v42.42,23.75 42.16,23.75
  Bottom 1.016: v15.37,4.19 27.56,4.19 v29.46,6.1 | 42.16,23.75 v37.72,19.3
N$50
  Top 0.254: LED_DRIVER.19 74.35,25.98 75.56,24.76 85.85,24.76 91.57,19.05 R17.1
N$51
  Top 0.254: LED_DRIVER.18 73.85,25.34 75.18,24 81.91,24 87.5,18.42 R16.1
N$52
  Top 0.305: C7.2
  Top 1.016: U$4.5 34.16,30.23 32.26,28.32 C7.2
N$53
  Top 0.305: LED_DRIVER.11 68.21,28.72 67.69,28.19 67.69,23.37 71.12,19.94 77.34,19.94 80.01,17.27 R9.2
N$54
  Top 0.305: LED_DRIVER.10 67.32,29.22 66.93,28.83 66.93,22.48 70.23,19.18 74.55,19.18 76.58,17.14 R8.2
N$55
  Top 0.305: LED_DRIVER.9 66.29,29.72 65.91,29.34 65.91,21.84 69.85,17.91 72.26,17.91 73.41,16.76 R7.2
N$56  (via drill 0.6 pad 0.25)
  Top 0.305: U$1.13 64.51,47.49 64.26,47.24 64.26,43.69 64.64,43.31 65.28,43.31 65.91,42.67 v65.91,35.31
  Bottom 0.254: v65.91,35.31 65.91,30.35 70.49,25.78 78.49,25.78 81.66,22.61
  Bottom 0.305: 81.66,22.61 90.17,14.1 RPI.6
N$58  (via drill 2.54)
  other vias: 120.27,3.05
N$59
  Top 0.254: LED_DRIVER.17 73.35,24.18 74.8,22.73 78.74,22.73 83.57,17.91 R10.1
N$60
  Top 0.305: U$1.57 102.79,51.99 106.81,56.01 BUTTONS.4
N$61  (via drill 2.54)
  other vias: 2.92,3.18
N$62
  Top 0.305: R16.2 87.5,12.45 83.44,8.38 LEDS.5
N$63
  Top 0.305: LCD.4 99.69,74.17 89.66,64.13 79.88,64.13 75.08,59.33 U$1.66
N$64
  Top 0.254: 64.09,32.72 63.63,32.26 R2.2
  Top 0.305: LED_DRIVER.3 64.09,32.72
N$65
  Top 0.305: R17.2 91.54,12.68 89.53,10.67 87.63,10.67 85.98,9.02 LEDS.4
N$66
  Top 0.305: R18.2 95.76,12.32 93.73,10.29 90.68,10.29 88.52,8.13 LEDS.3
N$67
  Top 0.305: R19.2 98.78,12.55 95.5,9.27 92.46,9.27 91.06,7.87 LEDS.2
N$68
  Top 0.305: R20.2 104.52,11.81 99.69,6.98 LEDS.1
N$70  (via drill 0.6)
  Top 0.305: U$1.75 70.58,57.88 72.77,60.07 72.77,73.53 v72.01,74.3 | v59.56,74.3 59.56,75.18 60.07,75.69 IC1.19
  Bottom 0.305: v72.01,74.3 v59.56,74.3
N$93
  Top 0.305: X6.2 8.23,56.01 R11.2
N$94
  Top 0.406: X6.1 R12.2
N$95
  Top 0.305: U$1.58 99.48,52.49 105.54,58.55 BUTTONS.3
N$96
  Top 0.305: U$1.56 107.5,51.49 109.47,53.47 BUTTONS.5
N$97
  Top 0.305: U$1.55 113.35,50.99 BUTTONS.6
N$99
  Top 0.305: IC2.3 12.73,53.72 R12.1
  Top 0.406: R12.1 R11.1 14.63,61.98 R13.2
N$100  (via drill 0.6)
  Top 0.305: IC2.6 22.73,53.72 v23.62,52.83 | v24.38,59.44 23.52,59.44 R13.1 25.15,61.98 27.18,64.01 31.39,64.01 R14.2 37.08,61.98 38.35,60.71 38.35,55.37 38.23,55.24 IC3.3
  Bottom 0.305: v23.62,52.83 24.38,52.83 24.89,53.34 24.89,58.93 v24.38,59.44
N$101  (via drill 0.6 pad 0.25)
  Top 0.305: IC3.6 27.3,55.24 26.16,56.39 26.16,57.56 R14.1 30.58,59.97 30.86,59.69 v35.94,59.69
  Bottom 0.305: v35.94,59.69 37.21,59.69 41.15,69.98 D2.A
N$102
  Bottom 0.305: R15.2 49.4,43.05
  Bottom 1.016: 49.4,43.05 49.4,45.34 44.83,49.91 D2.C
N$103  (via drill 0.6 pad 0.25)
  Top 0.305: U$1.23 68.98,40.53 v68.45,40
  Bottom 0.305: R15.1 55.98,39.34 56.51,39.88 68.33,39.88 v68.45,40
  Bottom 1.016: R15.1 45.74,39.34 44.32,40.77 C12.1
RPI  (via drill 0.6)
  Top 0.305: U$1.46 85.84,46.49 v86.23,46.48 86.36,46.48 108.58,24.26 RPI.2
  Bottom 0.305: LCD.6 104.78,73.15 89.28,57.66 89.28,46.86 88.9,46.48 v86.23,46.48
V+
  Top 0.305: IC2.7 25.02,54.99 26.16,53.85 29.02,53.85 IC3.7
V-  (via drill 0.6 pad 0.25)
  Top 0.305: IC3.4 34.35,58.23 34.04,58.55 32.51,58.55 v31.88,57.91 | v21.46,49.28 18.86,49.28 IC2.4
  Bottom 0.305: v31.88,57.91 31.88,50.16 30.99,49.28 v21.46,49.28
